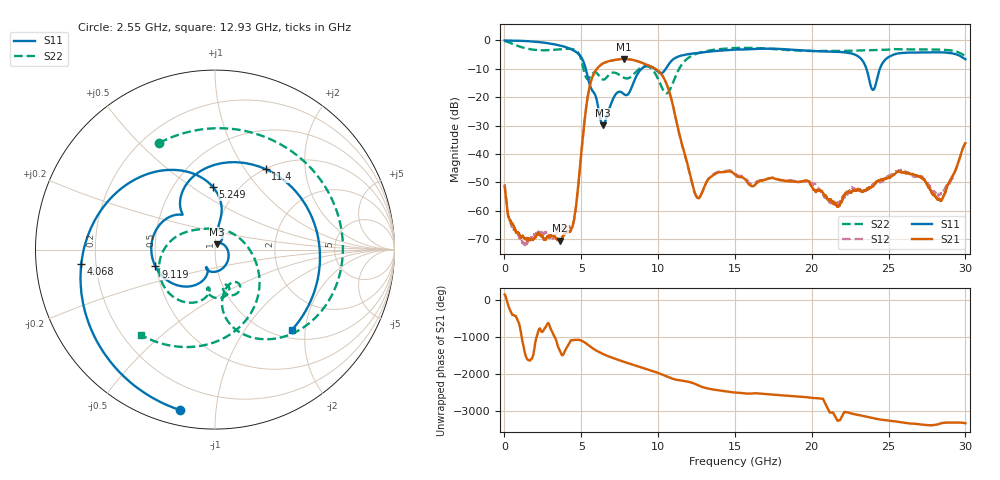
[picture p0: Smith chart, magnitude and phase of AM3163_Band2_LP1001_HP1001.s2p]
!Agilent Technologies,E8364B,MY43040894,A.07.50.67
!Agilent E8364B: A.07.50.67
!Date: Thursday, August 20, 2020 11:14:38
!Correction: S11(Full 2 Port(1,2))
!S21(Full 2 Port(1,2))
!S12(Full 2 Port(1,2))
!S22(Full 2 Port(1,2))
!S2P File: Measurements: S11, S21, S12, S22:
# Hz S  dB  R 50
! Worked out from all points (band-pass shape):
!   3201 points, 10 MHz to 30 GHz, reference 50 ohm
!   highest |S21| = -6.53 dB at 7.798 GHz (marker M1); lowest = -70.5 dB at 3.628 GHz (marker M2)
!   |S21| within 3 dB of the highest: 6.089 GHz to 9.678 GHz (3.589 GHz wide, 45.5 % of centre)
!   lowest |S11| = -29.8 dB at 6.43 GHz (marker M3), VSWR 1.07, Z = 51.1 + j3.07 ohm
!   |S11| at or under -10 dB: 5.291 GHz to 8.918 GHz (3.627 GHz wide, 51.1 % of centre); 9.773 GHz to 10.5 GHz (727.6 MHz wide, 7.18 % of centre); 23.56 GHz to 24.43 GHz (872.3 MHz wide, 3.64 % of centre)
!   |S22| runs from -18.6 to -0.2 dB; largest |S21 - S12| = 0.0048
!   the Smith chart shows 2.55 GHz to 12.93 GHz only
!   S11 on the Smith chart (normalised r, x): 2.55 GHz: 0.07, -0.80; 4.068 GHz: 0.14, -0.05; 5.249 GHz: 0.77, +0.61; 9.119 GHz: 0.49, -0.11; 11.4 GHz: 1.01, +1.25; 12.93 GHz: 1.16, -1.69
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1e7  -0.00 -2.7  -51.46 135.9  -50.66 42.9  -0.21 -9.2
6.285438e8  -0.08 -24.6  -65.66 -64.2  -66.34 -69.6  -1.44 -78.8
1.331434e9  -0.21 -52.5  -69.90 1.6  -72.51 99.9  -2.70 -148.4
2.549778e9  -0.77 -102.2  -69.85 -94.6  -67.97 109.3  -3.47 117.6
3.627544e9  -1.81 -150.7  -70.52 50.9  -66.21 -133.9  -3.11 43.8
4.068022e9  -2.50 -173.8  -67.33 159.9  -65.39 3.3  -2.94 12.1
5.014581e9  -6.09 116.6  -38.80 -23.7  -38.99 -24.4  -7.15 -77.4
5.248878e9  -9.16 91.8  -26.62 -78.8  -26.62 -79.0  -12.23 -78.2
6.429734e9  -29.85 68.8  -8.05 -23.8  -8.07 -23.9  -13.81 -74.0
7.798028e9  -19.01 -116.7  -6.53 125.7  -6.56 125.7  -13.21 -101.2
9.119462e9  -9.25 -164.2  -8.23 -48.2  -8.24 -48.3  -9.09 -131.7
1.000979e10  -11.11 135.5  -10.72 -171.8  -10.72 -171.8  -13.73 154.6
1.139683e10  -5.52 57.8  -33.33 -8.4  -33.57 -9.8  -9.74 -40.8
1.293382e10  -4.16 -46.4  -52.73 164.1  -52.50 167.2  -4.01 -131.1
1.5005e10  -3.26 -140.0  -47.33 22.4  -46.88 23.4  -2.67 150.9
1.777908e10  -2.95 95.8  -48.93 -42.3  -48.92 -44.9  -3.14 43.3
2.000958e10  -3.71 -18.3  -51.53 -121.2  -50.42 -115.8  -3.73 -39.8
2.284926e10  -5.09 -139.2  -52.71 154.4  -52.65 152.0  -3.57 -122.7
2.398326e10  -17.44 -142.4  -51.41 58.2  -50.99 61.1  -3.40 -151.1
2.500479e10  -5.85 -135.7  -48.44 -10.4  -47.67 -9.8  -3.24 -175.6
2.837867e10  -4.20 107.6  -56.64 -89.8  -53.96 -98.4  -3.25 96.7
3e10  -6.62 46.8  -36.22 -80.0  -36.11 -79.1  -5.49 47.9
